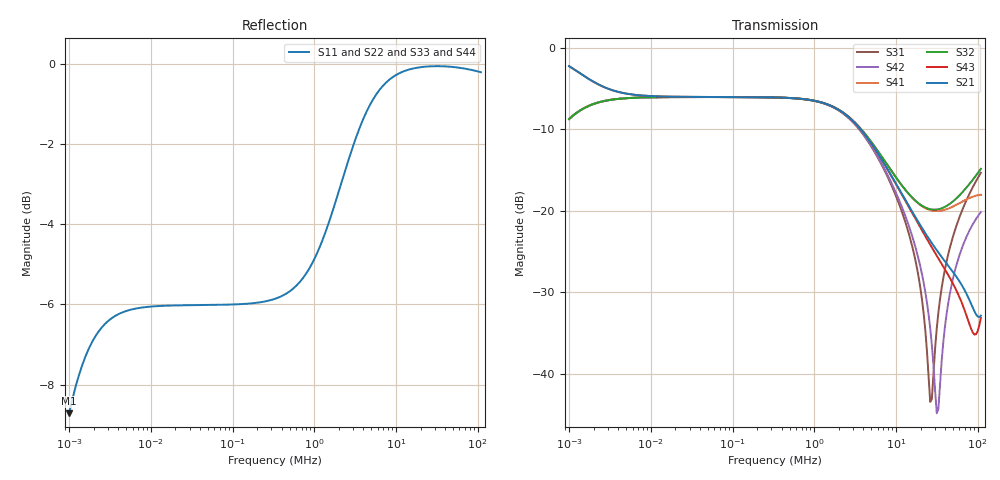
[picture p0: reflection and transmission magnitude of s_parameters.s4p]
! EM Consulting and Software
! Touchstone file was created on 2026-03-09  16:25:52
# HZ S RI R 50.0000
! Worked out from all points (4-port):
!   253 points, 1 kHz to 109.6 MHz, reference 50 ohm
!   strongest paths, dB at 1 kHz, 18.2 kHz, 331.1 kHz, 6.026 MHz, 109.6 MHz:
!     S21: -2.2, -6.0, -6.1, -13.0, -32.9
!     S43: -2.2, -6.0, -6.1, -13.0, -33.1
!     S32: -8.7, -6.0, -6.1, -12.7, -14.8
!     S41: -8.7, -6.0, -6.1, -12.7, -18.0
!     S42: -8.7, -6.0, -6.1, -13.4, -20.2
!     S31: -8.7, -6.0, -6.1, -13.5, -15.3
!   lowest |S11| = -8.7 dB at 1 kHz (marker M1), VSWR 2.16, Z = 72.5 + j41.8 ohm
!   |S11| at or under -10 dB: nowhere
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1000  0.2686 0.2494  0.7314 -0.2494  0.2685 0.2491  -0.2685 -0.2491
      0.7314 -0.2494  0.2686 0.2494  -0.2685 -0.2491  0.2685 0.2491
      0.2685 0.2491  -0.2685 -0.2491  0.2687 0.2494  0.7313 -0.2494
      -0.2685 -0.2491  0.2685 0.2491  0.7313 -0.2494  0.2687 0.2494
2290868  0.6861 0.2356  0.3142 -0.2441  0.3137 -0.2384  -0.314 0.2469
         0.3142 -0.2441  0.6854 0.2361  -0.314 0.2469  0.3144 -0.2389
         0.3137 -0.2384  -0.314 0.2469  0.6863 0.2354  0.3139 -0.2439
         -0.314 0.2469  0.3144 -0.2389  0.3139 -0.2439  0.6857 0.2359
1.380384e7  0.9805 0.0567  0.0177 -0.1098  0.0189 -0.0756  -0.017 0.1287
            0.0177 -0.1098  0.9792 0.0645  -0.017 0.1289  0.0201 -0.0836
            0.0189 -0.0756  -0.017 0.1289  0.9808 0.0546  0.0173 -0.108
            -0.017 0.1287  0.0201 -0.0836  0.0173 -0.108  0.9796 0.0629
2.630268e7  0.9921 -0.0335  -0.000687 -0.0655  0.0064 -0.00201  0.00222 0.101
            -0.000687 -0.0655  0.9921 -0.0189  0.0024 0.1023  0.00615 -0.0179
            0.0064 -0.00201  0.0024 0.1023  0.992 -0.0384  -0.000834 -0.0619
            0.00222 0.101  0.00615 -0.0179  -0.000834 -0.0619  0.9925 -0.0212
3.162278e7  0.9913 -0.0602  -0.00382 -0.0572  0.00671 0.0178  0.00584 0.0995
            -0.00382 -0.0572  0.9921 -0.0431  0.0062 0.1017  0.00552 -0.00148
            0.00671 0.0178  0.0062 0.1017  0.9909 -0.0666  -0.00383 -0.0529
            0.00584 0.0995  0.00552 -0.00148  -0.00383 -0.0529  0.9925 -0.0452
4.786301e7  0.9832 -0.1254  -0.0104 -0.0421  0.013 0.0633  0.0142 0.1043
            -0.0104 -0.0421  0.9867 -0.1029  0.0158 0.1112  0.00791 0.0339
            0.013 0.0633  0.0158 0.1112  0.981 -0.1386  -0.00983 -0.0358
            0.0142 0.1043  0.00791 0.0339  -0.00983 -0.0358  0.9877 -0.1023
1.096478e8  0.9331 -0.2863  -0.0225 0.0036  0.0565 0.1617  0.0329 0.121
            -0.0225 0.0036  0.9399 -0.2702  0.058 0.1715  0.0245 0.0951
            0.0565 0.1617  0.058 0.1715  0.9022 -0.3475  -0.0168 0.0143
            0.0329 0.121  0.0245 0.0951  -0.0168 0.0143  0.9594 -0.2304
